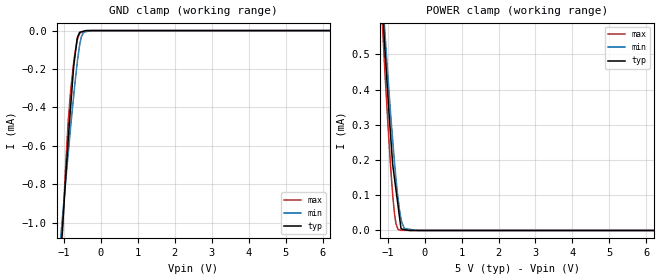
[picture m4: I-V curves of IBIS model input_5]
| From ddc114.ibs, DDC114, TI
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|   input_5 Model
[Model]   input_5
Model_type   Input
Vinl = 1
Vinh = 4
|   typ   min   max
|   (nom PVT)   (fast PVT)   (slow PVT)
|C_comp from frequency sweep method (F=19.2MHz)
|Average
C_comp   4.786e-13   4.166e-13   5.402e-13
|C_comp from LC tank measurement(L=1nH)
|Average
|Resonant Frequency(Hz)   5.930e+10   6.309e+10   4.449e+10
|C_comp   7.210e-15   6.370e-15   1.281e-14
| Where nom  PVT is Nominal Process, 5V, 27C
|   Fast PVT is Strong Process,  5.25V, -40C
|   Slow PVT is Weak Process,   4.75V, 87C
[Model Spec]
|Subparameter   typ   min   max
Vinl   1.0   0.95   1.05
Vinh   4.0   3.8   4.2
[Voltage Range]   5   4.75   5.25
|Ambient Temperature   25   85   -40
|Junction Temperature
[Temperature Range]   27   87   -40
[Power Clamp Reference]   5   4.75   5.25
[GND Clamp Reference]   0   0   0
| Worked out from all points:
|   GND clamp passes 1 mA (typ) near -1.03 V on its own axis
|   POWER clamp passes 1 mA (typ) near -1.35 V on its own axis
[GND Clamp]
|   Voltage   I(typ)   I(min)   I(max)
-5V       -13.86mA   -10.07mA   -20.07mA
-1.08V    -1.151mA   -1.06mA    -1.23mA
-1.04V    -1.029mA   -972uA     -1.053mA
-955.5mV  -776.7uA   -790.2uA   -714.9uA
-892.5mV  -594.8uA   -657.1uA   -498.9uA
-819mV    -398.3uA   -503.8uA   -313uA
-735mV    -184.4uA   -338.2uA   -165.1uA
-640mV    -38.79uA   -167.5uA   -52.15uA
-570mV    -8.716uA   -69.57uA   -14.18uA
-470.3mV  -3.227uA   -9.296uA   -5.622uA
-270.7mV  -67.14nA   -41.41nA   -32.51nA
10V       0A         0A         0A
[POWER Clamp]
|   Voltage   I(typ)   I(min)   I(max)
-5V       8.313mA    7.74mA     9.072mA
-1.306V   927.2uA    940uA      908.6uA
-1.088V   537.3uA    582.2uA    475.8uA
-1.076V   517.7uA    564.4uA    453.1uA
-992.2mV  379.6uA    436.4uA    300.2uA
-865mV    187.9uA    257.1uA    102.9uA
-813.7mV  146.6uA    190.2uA    46.31uA
-719.2mV  70.27uA    91.86uA    3.24uA
-640.5mV  6.702uA    35.52uA    144.4nA
-546.3mV  2.619uA    5.482uA    123.2nA
-190mV    0A         0A         42.85nA
10V       0A         0A         0A
